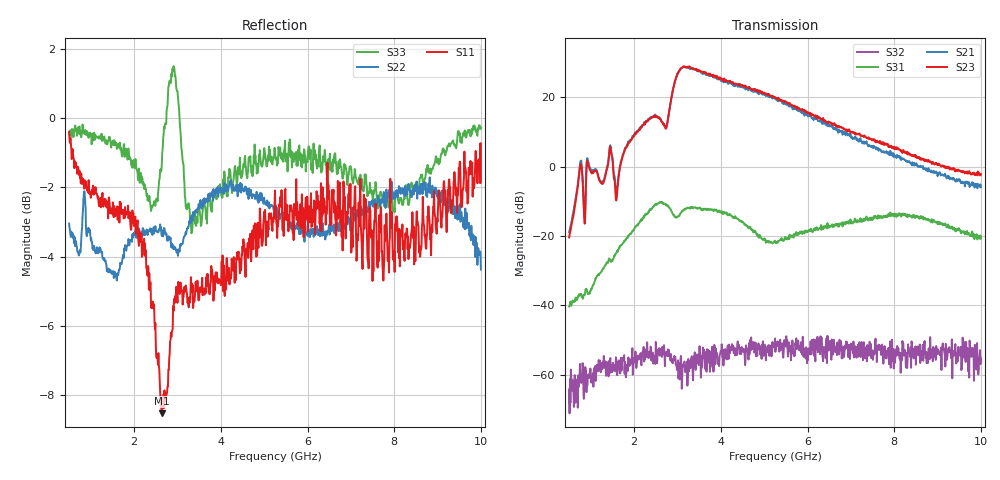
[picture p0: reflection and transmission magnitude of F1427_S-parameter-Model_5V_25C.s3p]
!Keysight Technologies,N5242B,MY57041011,A.15.65.19
!Date: Tuesday, September 26, 2023 12:02:05
!Correction: S11(C  3-Port  )
!S12(C  3-Port  )
!S13(C  3-Port  )
!S21(C  3-Port  )
!S22(C  3-Port  )
!S23(C  3-Port  )
!S31(C  3-Port  )
!S32(C  3-Port  )
!S33(C  3-Port  )
!S3P File: Measurements: <S11,S12,S13>,
!<S21,S22,S23>,
!<S31,S32,S33>:
# Hz S  RI  R 50
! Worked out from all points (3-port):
!   951 points, 500 MHz to 10 GHz, reference 50 ohm
!   strongest paths, dB at 500 MHz, 2.87 GHz, 5.25 GHz, 7.63 GHz, 10 GHz:
!     S23: -20.5, 20.4, 19.8, 7.0, -2.2
!     S21: -18.9, 20.6, 19.9, 5.3, -6.0
!     S31: -40.4, -13.1, -21.4, -14.1, -20.7
!     S32: -64.3, -56.3, -49.6, -51.9, -55.3
!   lowest |S11| = -8.5 dB at 2.64 GHz (marker M1), VSWR 2.20, Z = 28.9 + j22.3 ohm
!   |S11| at or under -10 dB: nowhere
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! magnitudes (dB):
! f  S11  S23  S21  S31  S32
! 500 MHz  -0.4  -20.5  -18.9  -40.4  -64.3
! 760 MHz  -1.7  0.4  1.5  -36.8  -61.5
! 970 MHz  -2.2  -0.7  0.0  -36.4  -60.6
! 1.15 GHz  -2.2  -1.9  -1.7  -31.6  -57.4
! 1.43 GHz  -2.4  4.3  4.9  -26.7  -59.7
! 1.6 GHz  -2.8  -8.8  -7.6  -24.7  -59.4
! 2.64 GHz  -8.5  12.8  12.8  -10.5  -54.9
! 3.14 GHz  -5.2  28.9  28.7  -12.5  -57.4
! 5.25 GHz  -2.1  19.8  19.9  -21.4  -49.6
! 10 GHz  -1.9  -2.2  -6.0  -20.7  -55.3
